TYPE E_AnalysisIDs :
(
	(* Source Ids *)
	eID_Source1 := 1,
	eID_Source2,
	eID_Source3,
	eID_Source4,
	eID_Source5,
	eID_Source6,
	(* Spectrum Ids for each channel *)
	eID_Spectrum1,
	eID_Spectrum2,
	eID_Spectrum3,
	eID_Spectrum4,
	eID_Spectrum5,
	eID_Spectrum6,
	(* Sink Ids for each channel *)
	eID_Sink1,
	eID_Sink2,
	eID_Sink3,
	eID_Sink4,
	eID_Sink5,
	eID_Sink6
) UDINT;
END_TYPE
